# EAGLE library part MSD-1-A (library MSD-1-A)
Memory Card Connectors 9 Positions, Push In, Auto Eject Out, SMT, 1.8 mm Height Above Board, Source: Datasheet
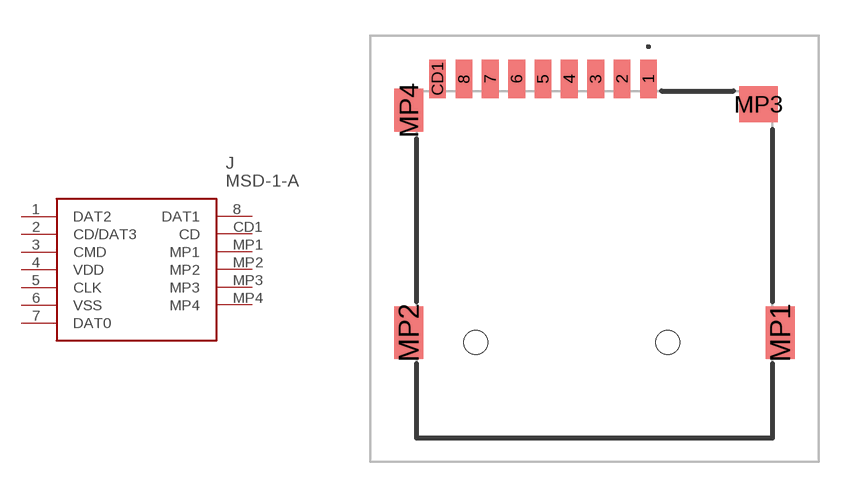
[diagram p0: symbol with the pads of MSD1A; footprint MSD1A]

Designator prefix J

## MSD-1-A (Description: Memory Card Connectors 9 Positions, Push In, Auto Eject Out, SMT, 1.8 mm Height Above Board,; Height: 2mm; Manufacturer_Name: CUI Devices; Manufacturer_Part_Number: MSD-1-A; Mouser_Part_Number: 179-MSD-1-A; Mouser_Price-Stock: https://www.mouser.co.uk/ProductDetail/CUI-Devices/MSD-1-A?qs=Z%252BL2brAPG1Ip18XLC4tUPQ%3D%3D)  [MSD1A]
1  DAT2
2  CD/DAT3
3  CMD
4  VDD
5  CLK
6  VSS
7  DAT0
8  DAT1
CD1  CD
MP1  MP1
MP2  MP2
MP3  MP3
MP4  MP4

## Footprint MSD1A (pad centres in mm)
MSD-1-A-1
smd 0.7 x 1.6: 1 2.25,7.5; 2 1.15,7.5; 3 0.05,7.5; 4 -1.05,7.5; 5 -2.15,7.5; 6 -3.25,7.5; 7 -4.35,7.5; 8 -5.45,7.5; CD1 -6.55,7.5
smd 1.2 x 2.2: MP1 7.75,-3.1; MP2 -7.75,-3.1
smd 1.6 x 1.5: MP3 6.85,6.45
smd 1.2 x 1.8: MP4 -7.75,6.2
hole 1 at 3.05,-3.5
hole 1 at -4.95,-3.5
